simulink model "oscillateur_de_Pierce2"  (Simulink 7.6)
settings: Solver=ode15s  StartTime=0.0  StopTime=0.05  RelTol=1e-3
InitFcn:
  | clc
libraries: fl_lib x9, elec_lib x3, nesl_utility x3

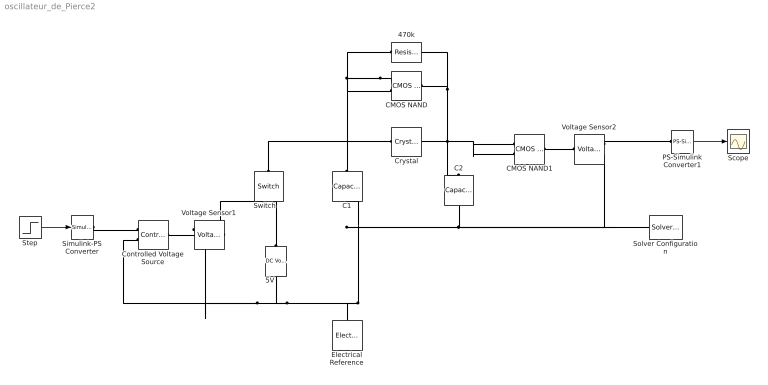
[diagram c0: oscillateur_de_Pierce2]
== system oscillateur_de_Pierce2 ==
  470k : fl_lib/Electrical/Electrical Elements/Resistor  DialogController=NetworkEngine.DynNeDlgSource  SystemSampleTime=-1  R=470 kOhm  i_Log=off  v_Log=off  LocalVarNames=|i|v  LocalVarDescs=|i|v  LocalVarLogging=[0 0]
  5V : fl_lib/Electrical/Electrical Sources/DC Voltage Source  DialogController=NetworkEngine.DynNeDlgSource  SystemSampleTime=-1  v0=5 V  i_Log=off  v_Log=off  LocalVarNames=|i|v  LocalVarDescs=|i|v  LocalVarLogging=[0 0]
  C1 : fl_lib/Electrical/Electrical Elements/Capacitor  DialogController=NetworkEngine.DynNeDlgSource  SystemSampleTime=-1  c=10 nF  v0=0 V  r=1e-6 Ohm  g=0 1/Ohm  i_Log=off  v_Log=off  vc_Log=off  LocalVarNames=|i|v|vc  LocalVarDescs=|i|v|Internal variable for voltage across capacitor term  LocalVarLogging=[0 0 0]
  C2 : fl_lib/Electrical/Electrical Elements/Capacitor  DialogController=NetworkEngine.DynNeDlgSource  SystemSampleTime=-1  c=10 nF  v0=0 V  r=1e-6 Ohm  g=0 1/Ohm  i_Log=off  v_Log=off  vc_Log=off  LocalVarNames=|i|v|vc  LocalVarDescs=|i|v|Internal variable for voltage across capacitor term  LocalVarLogging=[0 0 0]
  CMOS NAND : elec_lib/Integrated Circuits/Logic/CMOS NAND  DialogController=NetworkEngine.DynNeDlgSource  SystemSampleTime=-1  V_IL=2 V  V_IH=3 V  C_IN=5 pF  output_type=1  V_OL=0 V  V_OH=5 V  V_CC=5 V  V_meas=5 V  R_OUT=25 Ohm  R_OH=[ 25 250 ] Ohm  I_OH=63 mA  R_OL=[ 30 800 ] Ohm  I_OL=-45 mA  Delay=25 ns  Ron=5 Ohm  Vf=0.6 V  output_state=1  LocalVarLogging=[]
  CMOS NAND1 : elec_lib/Integrated Circuits/Logic/CMOS NAND  DialogController=NetworkEngine.DynNeDlgSource  SystemSampleTime=-1  V_IL=2 V  V_IH=3 V  C_IN=5 pF  output_type=1  V_OL=0 V  V_OH=5 V  V_CC=5 V  V_meas=5 V  R_OUT=25 Ohm  R_OH=[ 25 250 ] Ohm  I_OH=63 mA  R_OL=[ 30 800 ] Ohm  I_OL=-45 mA  Delay=25 ns  Ron=5 Ohm  Vf=0.6 V  output_state=1  LocalVarLogging=[]
  Controlled Voltage Source : fl_lib/Electrical/Electrical Sources/Controlled Voltage Source  DialogController=NetworkEngine.DynNeDlgSource  SystemSampleTime=-1  i_Log=off  v_Log=off  LocalVarNames=|i|v  LocalVarDescs=|i|v  LocalVarLogging=[0 0]
  Crystal : elec_lib/Passive Devices/Crystal  DialogController=NetworkEngine.DynNeDlgSource  SystemSampleTime=-1  param=1  L1=6.742e+3 H  Fs=100 kHz  Fa=32.768 kHz  param_R1=1  R1=15 kOhm  Q=9e+4  C1=0.0035 pF  CL=12.5 pF  C0=1.6 pF  V_ini=0 V  LocalVarLogging=[]
  Electrical Reference : fl_lib/Electrical/Electrical Elements/Electrical Reference  DialogController=NetworkEngine.DynNeDlgSource  SystemSampleTime=-1  i_Log=off  LocalVarNames=|i  LocalVarDescs=|i  LocalVarLogging=0
  PS-Simulink Converter1 : nesl_utility/PS-Simulink Converter  DialogController=NetworkEngine.DynNeUtilDlgSource  SystemSampleTime=-1  PhysicalDomain=network_engine_domain  LeftPortType=input  RightPortType=output  SubClassName=ps_output  Unit=1  AffineConversion=off
  Scope : Scope
  Simulink-PS Converter : nesl_utility/Simulink-PS Converter  DialogController=NetworkEngine.DynNeUtilDlgSource  SystemSampleTime=-1  PhysicalDomain=network_engine_domain  LeftPortType=input  RightPortType=output  SubClassName=ps_input  Unit=1  AffineConversion=off  InputFilterTimeConstant=.001  UdotUserProvided=0
  Solver Configuration : nesl_utility/Solver Configuration  DialogController=NetworkEngine.DynNeUtilDlgSource  SystemSampleTime=-1  PhysicalDomain=network_engine_domain  LeftPortType=input  RightPortType=generic  SubClassName=solver  Accelerate=off  Profile=off  ResidualTolerance=1e-9  MaxNonlinIter=3  MaxModeIter=2  DoFixedCost=off  UseLocalSampling=off  DoDC=off  LinearAlgebra=Sparse  LocalSolverSampleTime=.001  LocalSolverChoice=NE_BACKWARD_EULER_ADVANCER  UseLocalSolver=off
  Step : Step  Time=0.02  Before=1  After=0  SampleTime=0
  Switch : fl_lib/Electrical/Electrical Elements/Switch  DialogController=NetworkEngine.DynNeDlgSource  SystemSampleTime=-1  R_closed=0.01 Ohm  G_open=1e-8 1/Ohm  Threshold=0  i_Log=off  v_Log=off  LocalVarNames=|i|v  LocalVarDescs=|i|v  LocalVarLogging=[0 0]
  Voltage Sensor1 : fl_lib/Electrical/Electrical Sensors/Voltage Sensor  DialogController=NetworkEngine.DynNeDlgSource  SystemSampleTime=-1  i1_Log=off  v1_Log=off  LocalVarNames=|i1|v1  LocalVarDescs=|i1|v1  LocalVarLogging=[0 0]
  Voltage Sensor2 : fl_lib/Electrical/Electrical Sensors/Voltage Sensor  DialogController=NetworkEngine.DynNeDlgSource  SystemSampleTime=-1  i1_Log=off  v1_Log=off  LocalVarNames=|i1|v1  LocalVarDescs=|i1|v1  LocalVarLogging=[0 0]
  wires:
  PS-Simulink Converter1/1 -> Scope/1
  Step/1 -> Simulink-PS Converter/1
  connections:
  Controlled Voltage Source/LConn1 -- Voltage Sensor1/LConn1
  Simulink-PS Converter/RConn1 -- Controlled Voltage Source/RConn1
  CMOS NAND/RConn1 -- C2/LConn1 -- Crystal/RConn1 -- CMOS NAND1/LConn1 -- CMOS NAND1/LConn2 -- 470k/RConn1
  CMOS NAND/LConn1 -- CMOS NAND/LConn2 -- C1/LConn1 -- Crystal/LConn1 -- Switch/LConn1 -- 470k/LConn1
  CMOS NAND1/RConn1 -- Voltage Sensor2/LConn1
  Controlled Voltage Source/RConn2 -- 5V/RConn1 -- Electrical Reference/LConn1 -- C1/RConn1 -- C2/RConn1 -- Voltage Sensor2/RConn2 -- Solver Configuration/RConn1 -- Voltage Sensor1/RConn2
  Voltage Sensor2/RConn1 -- PS-Simulink Converter1/LConn1
  5V/LConn1 -- Switch/RConn2
  Voltage Sensor1/RConn1 -- Switch/RConn1
